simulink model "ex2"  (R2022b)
settings: Solver=ode45  StartTime=0.0  StopTime=10.0  RelTol=1e-3  EnableMultiTasking=on

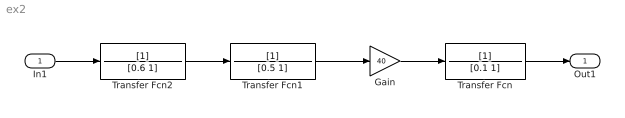
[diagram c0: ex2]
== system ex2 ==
  In1 : Inport
  Gain : Gain  Gain=40
  Transfer Fcn : TransferFcn  Denominator=[0.1 1]
  Transfer Fcn1 : TransferFcn  Denominator=[0.5 1]
  Transfer Fcn2 : TransferFcn  Denominator=[0.6 1]
  Out1 : Outport
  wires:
  Transfer Fcn/1 -> Out1/1
  Transfer Fcn1/1 -> Gain/1
  Gain/1 -> Transfer Fcn/1
  In1/1 -> Transfer Fcn2/1
  Transfer Fcn2/1 -> Transfer Fcn1/1
